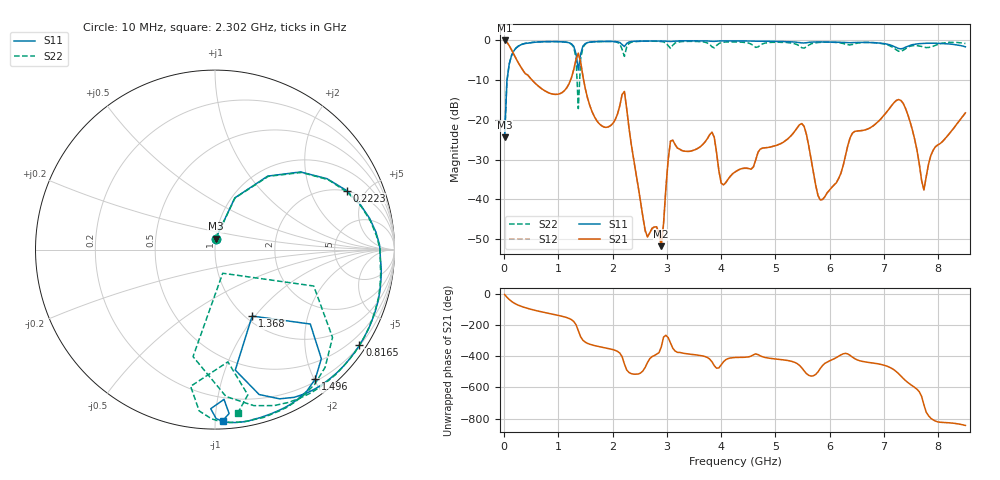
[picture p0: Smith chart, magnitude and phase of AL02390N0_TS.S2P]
!AVX CORPORATION
!PART NUMBER AL02390N0_TS
!DESCRIPTION: AIR CORE INDUCTOR, 90nH, 9 TURNS
!Agilent Technologies,E5071C,MY46102230,A.09.54
!Date: Mon Sep 03 16:43:30 2012
!Data & Calibration Information:
!Freq	S11:SOLT2(ON)	S21:SOLT2(ON)	S12:SOLT2(ON)	S22:SOLT2(ON)
# Hz S dB R 50
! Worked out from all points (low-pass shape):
!   201 points, 10 MHz to 8.5 GHz, reference 50 ohm
!   highest |S21| = -0.01 dB at 10 MHz (marker M1); lowest = -51.8 dB at 2.897 GHz (marker M2)
!   |S21| within 3 dB of the highest: start of sweep to 160.8 MHz
!   lowest |S11| = -24.4 dB at 10 MHz (marker M3), VSWR 1.13, Z = 50 + j6.07 ohm
!   |S11| at or under -10 dB: start of sweep to 54.69 MHz
!   |S22| runs from -24.3 to -0.2 dB; largest |S21 - S12| = 0.0049
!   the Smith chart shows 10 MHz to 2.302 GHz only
!   S11 on the Smith chart (normalised r, x): 10 MHz: 1.00, +0.12; 222.2 MHz: 1.97, +3.67; 816.5 MHz: 0.21, -3.31; 1.368 GHz: 1.07, -0.97; 1.496 GHz: 0.23, -2.02; 2.302 GHz: 0.05, -1.04
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1e7  -24.35 86.5  -0.01 -4.1  -0.05 -4.1  -24.29 86.8
5.245e7  -10.22 69.1  -0.45 -20.9  -0.43 -20.9  -10.21 68.8
2.2225e8  -1.90 24.2  -4.63 -65.8  -4.61 -65.9  -1.89 23.4
8.1655e8  -0.31 -33.5  -13.17 -124.3  -13.16 -124.4  -0.29 -36.7
1.2835e9  -1.47 -73.1  -7.36 -176.6  -7.36 -176.6  -1.72 -85.7
1.3684e9  -7.45 -60.8  -3.23 124.6  -3.23 124.5  -17.17 -72.0
1.4533e9  -1.42 -45.7  -9.04 62.7  -9.04 62.7  -1.75 -36.8
1.49575e9  -0.80 -52.3  -12.10 50.6  -12.09 50.6  -0.93 -46.9
2.2174e9  -1.56 -86.6  -12.87 -89.6  -12.87 -89.6  -4.02 -83.4
2.3023e9  -0.41 -87.4  -22.09 -144.0  -22.09 -144.2  -0.76 -81.9
2.59945e9  -0.16 -98.5  -47.77 -111.6  -48.09 -112.1  -0.20 -97.3
2.85415e9  -0.16 -105.4  -48.69 -17.1  -48.64 -14.2  -0.25 -106.1
2.8966e9  -0.15 -106.5  -51.81 19.8  -51.49 17.9  -0.30 -107.9
3.0664e9  -0.27 -110.1  -25.35 44.8  -25.34 44.7  -1.99 -108.0
4.255e9  -0.12 -117.3  -33.15 -47.6  -33.17 -47.9  -0.37 -131.2
5.48605e9  -0.62 -137.0  -20.94 -114.4  -20.94 -114.4  -1.85 -157.0
5.6983e9  -0.41 -139.7  -33.07 -165.4  -33.21 -165.1  -0.71 -153.3
5.8681e9  -0.37 -143.6  -40.08 -99.4  -39.94 -100.6  -0.47 -157.6
7.09915e9  -1.08 -171.3  -17.16 -109.8  -17.16 -109.7  -1.32 -172.3
7.3963e9  -1.71 -167.1  -17.10 164.4  -17.08 164.4  -2.09 -159.3
7.7359e9  -0.74 -175.1  -37.65 8.5  -37.66 8.1  -1.69 -162.9
8.5e9  -1.60 163.2  -18.25 -123.5  -18.26 -123.6  -0.78 -168.8
